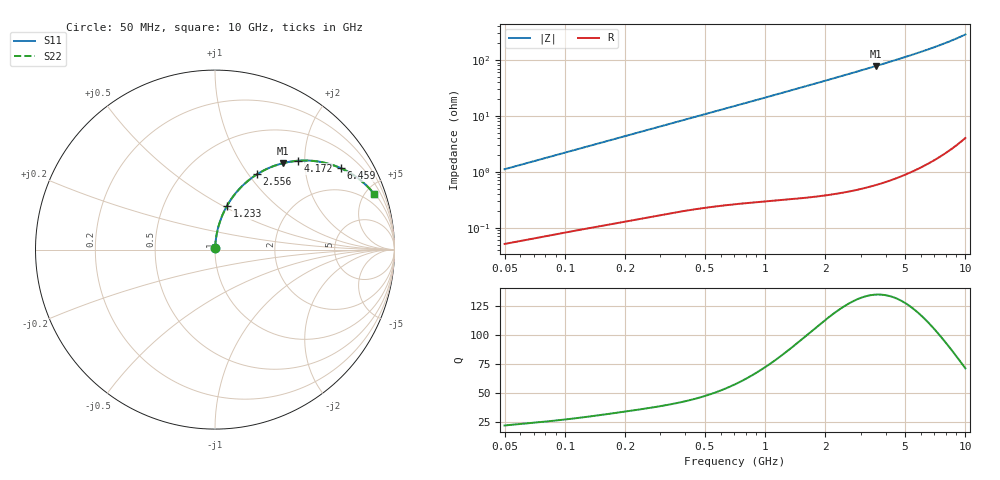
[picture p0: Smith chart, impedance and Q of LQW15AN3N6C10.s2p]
!Murata Part Number: LQW15AN3N6C10
!These Parameters are Measured in Series Mode Connection
!  o--[Z]--o
!Port1  Port2
!  o-------o
!Freq. Start=50[MHz] Stop=10[GHz], 401[Steps]
# Hz S RI R 50
!Freq.(Hz)	S 11(Real)	S 11(Imag)	S 21(Real)	S 21(Imag)	S 12(Real)	S 12(Imag)	S 22(Real)	S 22(Imag)
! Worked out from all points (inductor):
!   401 points, 50 MHz to 10 GHz, reference 50 ohm
!   read as one part in series: L = 3.52 nH near 51.34 MHz
!   highest Q = 135 at 3.559 GHz (marker M1), where L = 3.48 nH
!   S11 on the Smith chart (normalised r, x): 50 MHz: 1.00, +0.02; 1.233 GHz: 1.01, +0.52; 2.556 GHz: 1.01, +1.10; 4.172 GHz: 1.01, +1.85; 6.459 GHz: 1.03, +3.06; 10 GHz: 1.08, +5.73
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5e7  0.000635 0.0111  0.9994 -0.0111  0.9994 -0.0111  0.000635 0.0111
1.214486e8  0.00163 0.0265  0.9984 -0.0265  0.9984 -0.0265  0.00163 0.0265
1.956524e8  0.00305 0.0422  0.9969 -0.0422  0.9969 -0.0422  0.00305 0.0422
2.949953e8  0.00565 0.063  0.9943 -0.063  0.9943 -0.063  0.00565 0.063
4.689809e8  0.0121 0.0988  0.9879 -0.0988  0.9879 -0.0988  0.0121 0.0988
7.071068e8  0.0246 0.1464  0.9754 -0.1464  0.9754 -0.1464  0.0246 0.1464
9.589462e8  0.0424 0.1945  0.9576 -0.1945  0.9576 -0.1945  0.0424 0.1945
1.233369e9  0.0668 0.2438  0.9332 -0.2438  0.9332 -0.2438  0.0668 0.2438
1.465132e9  0.091 0.2824  0.909 -0.2824  0.909 -0.2824  0.091 0.2824
1.717543e9  0.1205 0.3207  0.8795 -0.3207  0.8795 -0.3207  0.1205 0.3207
2.095058e9  0.1693 0.3707  0.8307 -0.3707  0.8307 -0.3707  0.1693 0.3707
2.555552e9  0.2336 0.4192  0.7664 -0.4192  0.7664 -0.4192  0.2336 0.4192
2.99582e9  0.2972 0.4533  0.7028 -0.4533  0.7028 -0.4533  0.2972 0.4533
3.558764e9  0.3777 0.4811  0.6223 -0.4811  0.6223 -0.4811  0.3777 0.4811
4.171863e9  0.4605 0.4947  0.5395 -0.4947  0.5395 -0.4947  0.4605 0.4947
4.638213e9  0.5187 0.4958  0.4813 -0.4958  0.4813 -0.4958  0.5187 0.4958
5.156693e9  0.5777 0.49  0.4223 -0.49  0.4223 -0.49  0.5777 0.49
5.733131e9  0.6361 0.477  0.3639 -0.477  0.3639 -0.477  0.6361 0.477
6.458996e9  0.6996 0.454  0.3004 -0.454  0.3004 -0.454  0.6996 0.454
7.983737e9  0.8015 0.3936  0.1985 -0.3936  0.1985 -0.3936  0.8015 0.3936
9.114482e9  0.8554 0.3455  0.1446 -0.3455  0.1446 -0.3455  0.8554 0.3455
1e10  0.8881 0.3083  0.1119 -0.3083  0.1119 -0.3083  0.8881 0.3083
